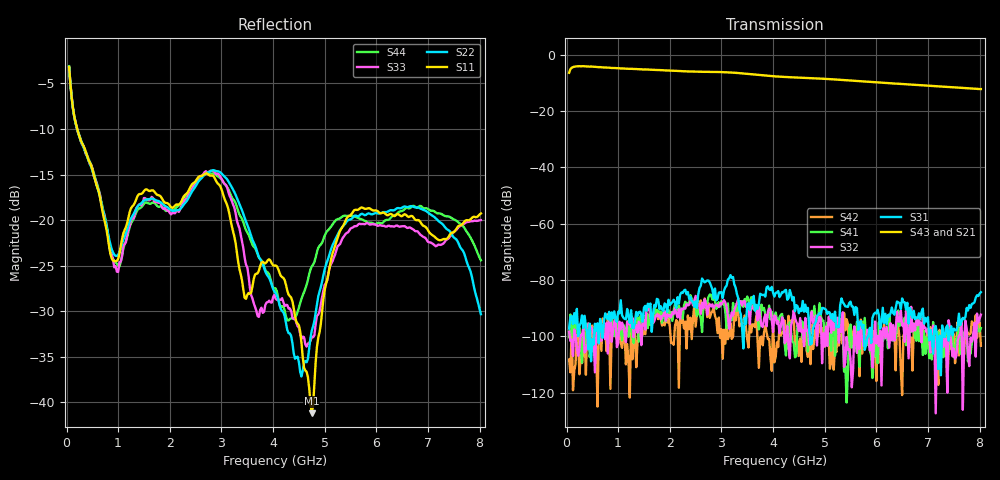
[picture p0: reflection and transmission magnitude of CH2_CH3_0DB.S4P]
!Agilent Technologies,E5071C,MY46316741,A.11.02
!Date: Thu May 28 14:37:49 2026
!Data & Calibration Information:
!1:CH2 INPUT 2:CH2 OUTPUT 3:CH3 INPUT 4:CH3 OUTPUT
!Freq	S11:SOLT4(ON)	S12:SOLT4(ON)	S13:SOLT4(ON)	S14:SOLT4(ON)
!	S21:SOLT4(ON)	S22:SOLT4(ON)	S23:SOLT4(ON)	S24:SOLT4(ON)
!	S31:SOLT4(ON)	S32:SOLT4(ON)	S33:SOLT4(ON)	S34:SOLT4(ON)
!	S41:SOLT4(ON)	S42:SOLT4(ON)	S43:SOLT4(ON)	S44:SOLT4(ON)
!PortZ  Port1:50+j0  Port2:50+j0  Port3:50+j0  Port4:50+j0
!Above PortZ is port z conversion or system Z0 setting when saving the data.
!When reading, reference impedance value at option line is always used.
# Hz S dB R 50
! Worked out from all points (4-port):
!   320 points, 50 MHz to 8.025 GHz, reference 50 ohm
!   strongest paths, dB at 50 MHz, 2.05 GHz, 4.05 GHz, 6.05 GHz, 8.025 GHz:
!     S43: -6.4, -5.7, -7.8, -9.9, -12.2
!     S21: -6.5, -5.8, -8.0, -10.1, -12.4
!     S31: -97.2, -87.8, -84.6, -92.6, -84.3
!     S32: -98.4, -91.4, -92.9, -103.4, -92.3
!     S41: -100.3, -94.5, -91.5, -95.0, -97.1
!     S42: -108.2, -102.3, -107.3, -103.0, -103.3
!   lowest |S11| = -41.2 dB at 4.75 GHz (marker M1), VSWR 1.02, Z = 50.3 + j0.824 ohm
!   |S11| at or under -10 dB: 207.7 MHz to end of sweep
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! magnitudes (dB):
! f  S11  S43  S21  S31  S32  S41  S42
! 50 MHz  -3.2  -6.4  -6.5  -97.2  -98.4  -100.3  -108.2
! 1 GHz  -24.2  -4.8  -5.0  -91.2  -102.5  -99.5  -98.7
! 2.85 GHz  -15.2  -6.2  -6.3  -86.5  -89.8  -87.0  -89.9
! 4.275 GHz  -27.7  -8.0  -8.2  -87.0  -96.3  -96.0  -103.6
! 4.75 GHz  -41.2  -8.4  -8.6  -102.5  -91.2  -90.9  -95.9
! 5.45 GHz  -19.6  -9.1  -9.3  -89.5  -104.7  -112.9  -95.5
! 8.025 GHz  -19.3  -12.2  -12.4  -84.3  -92.3  -97.1  -103.3
